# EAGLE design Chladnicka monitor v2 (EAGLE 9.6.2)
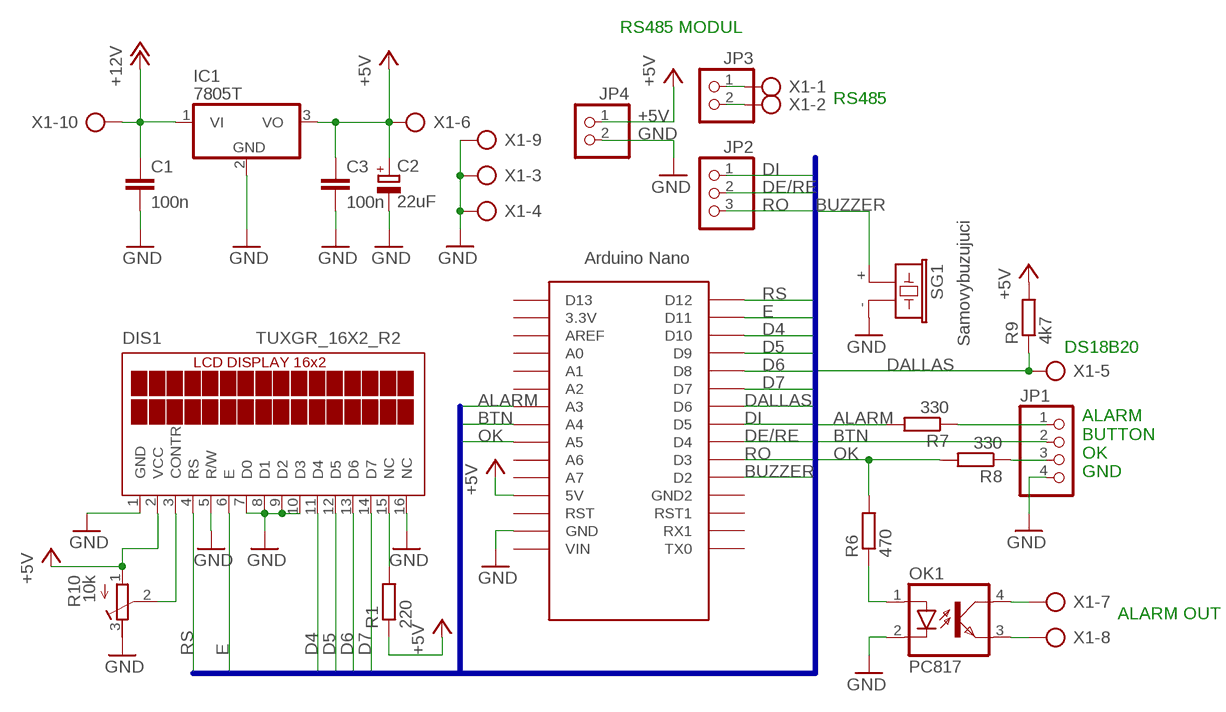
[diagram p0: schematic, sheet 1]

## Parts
C1  100n  C-EU050-024X044  [C050-024X044]
C2  22uF  CPOL-EUE2,5-6E  [E2,5-6E]
C3  100n  C-EU050-024X044  [C050-024X044]
DIS1  TUXGR_16X2_R2  [TUXGR_16X2_R2]
IC1  7805T  [TO220H]
JP1  PINHD-1X4  [1X04]
JP2  PINHD-1X3  [1X03]
JP3  PINHD-1X2  [1X02]
JP4  PINHD-1X2  [1X02]
OK1  PC817  [DIL04]
R1  220  R-EU_0204/7  [0204/7]
R6  470  R-EU_0204/7  [0204/7]
R7  330  R-EU_0204/7  [0204/7]
R8  330  R-EU_0204/7  [0204/7]
R9  4k7  R-EU_0204/7  [0204/7]
R10  10k  R-TRIMM3339P  [RTRIM3339P]
SG1  Samovybuzujuci  F/CM12P  [F/CM12P]
U$1  NANO  [NANO]
X1  AK500/10  [AK500/10]

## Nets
+5V: C2.+ C3.1 DIS1.2(VCC) IC1.3(VO) JP4.1 R1.1 R9.2 R10.1(A) U$1.5V X1.6
+12V: C1.1 IC1.1(VI) X1.10
ALARM: R7.2 U$1.A3
BTN: JP1.2 U$1.A4
BUZZER: SG1.+ U$1.D2
D4: DIS1.11(D4) U$1.D10
D5: DIS1.12(D5) U$1.D9
D6: DIS1.13(D6) U$1.D8
D7: DIS1.14(D7) U$1.D7
DALLAS: R9.1 U$1.D6 X1.5
DE/RE: JP2.2 U$1.D4
DI: JP2.1 U$1.D5
E: DIS1.6(E) U$1.D11
GND: C1.2 C2.- C3.2 DIS1.1(GND) DIS1.5(R/W) DIS1.7(D0) DIS1.8(D1) DIS1.9(D2) DIS1.10(D3) DIS1.16(NC) IC1.2(GND) JP1.4 JP4.2 OK1.2(C) R10.3(E) SG1.- U$1.GND X1.3 X1.4 X1.9
N$1: OK1.1(A) R6.1
N$2: JP1.3 R8.1
N$3: JP1.1 R7.1
N$4: JP3.2 X1.2
N$5: JP3.1 X1.1
N$6: DIS1.3(CONTR) R10.2(S)
N$7: OK1.4(COL) X1.7
N$8: OK1.3(EMIT) X1.8
N$10: DIS1.15(NC) R1.2
OK: R6.2 R8.2 U$1.A5
RO: JP2.3 U$1.D3
RS: DIS1.4(RS) U$1.D12
Unconnected: U$1.3.3V U$1.A0 U$1.A1 U$1.A2 U$1.A6 U$1.A7 U$1.AREF U$1.D13 U$1.GND1(GND2) U$1.ICSP1 U$1.ICSP2 U$1.ICSP3 U$1.ICSP4 U$1.ICSP5 U$1.ICSP6 U$1.RAW(VIN) U$1.RST U$1.RST1 U$1.RX1 U$1.TX0

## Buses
ALARM,BTN,BUZZER,D4,D5,D6,D7,DALLAS,DE/RE,DI,E,OK,RO,RS

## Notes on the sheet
- RS485 MODUL
- RS485
- DS18B20
- ALARM
  BUTTON
  OK
  GND
- ALARM OUT

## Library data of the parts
C1 C3 = rcl:C-EU: CAPACITOR, European symbol; SPICEPREFIX: C
C2 = rcl:CPOL-EU: POLARIZED CAPACITOR, European symbol; SPICEPREFIX: C
DIS1 = display-lcd:TUXGR_16X2_R2: Tuxgraphics LCD display 16x2 characters reflective, without background light Source: tuxgr_12x2_r2.pdf; OC_FARNELL: unknown; OC_NEWARK: unknown
IC1 = linear:78*: Positive VOLTAGE REGULATOR Source: http://cache.national.com/ds/LM/LM78L05.pdf http://www.fairchildsemi.com/ds/LM/LM7805.pdf
JP1 = pinhead:PINHD-1X4: PIN HEADER
JP2 = pinhead:PINHD-1X3: PIN HEADER
JP3 JP4 = pinhead:PINHD-1X2: PIN HEADER
OK1 = optocoupler:PC817: SHARP OPTO COUPLER; MPN: PC817X4J000F; OC_FARNELL: 9707727; OC_NEWARK: 97K7059
R1 R6-R9 = rcl:R-EU_: RESISTOR, European symbol; SPICEPREFIX: R
R10 = rcl:R-TRIMM: Trimm resistor; SPICEMODEL: X; SPICEPREFIXL: POT
SG1 = buzzer:F/CM12P: BUZZER; OC_FARNELL: unknown; OC_NEWARK: unknown
U$1 = Arduino-clone:NANO: Arduino Nano
X1 = con-ptr500:AK500/10: CONNECTOR; OC_FARNELL: unknown; OC_NEWARK: unknown

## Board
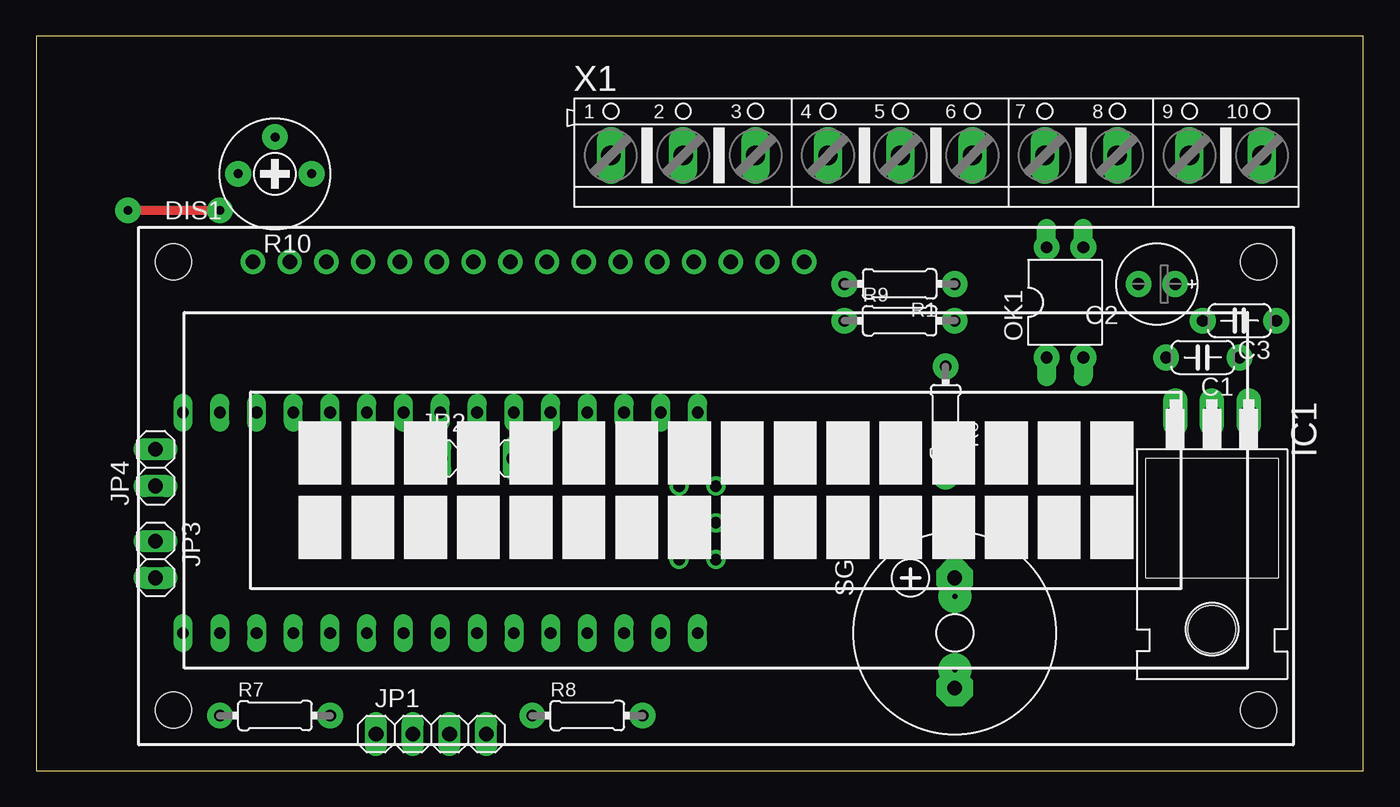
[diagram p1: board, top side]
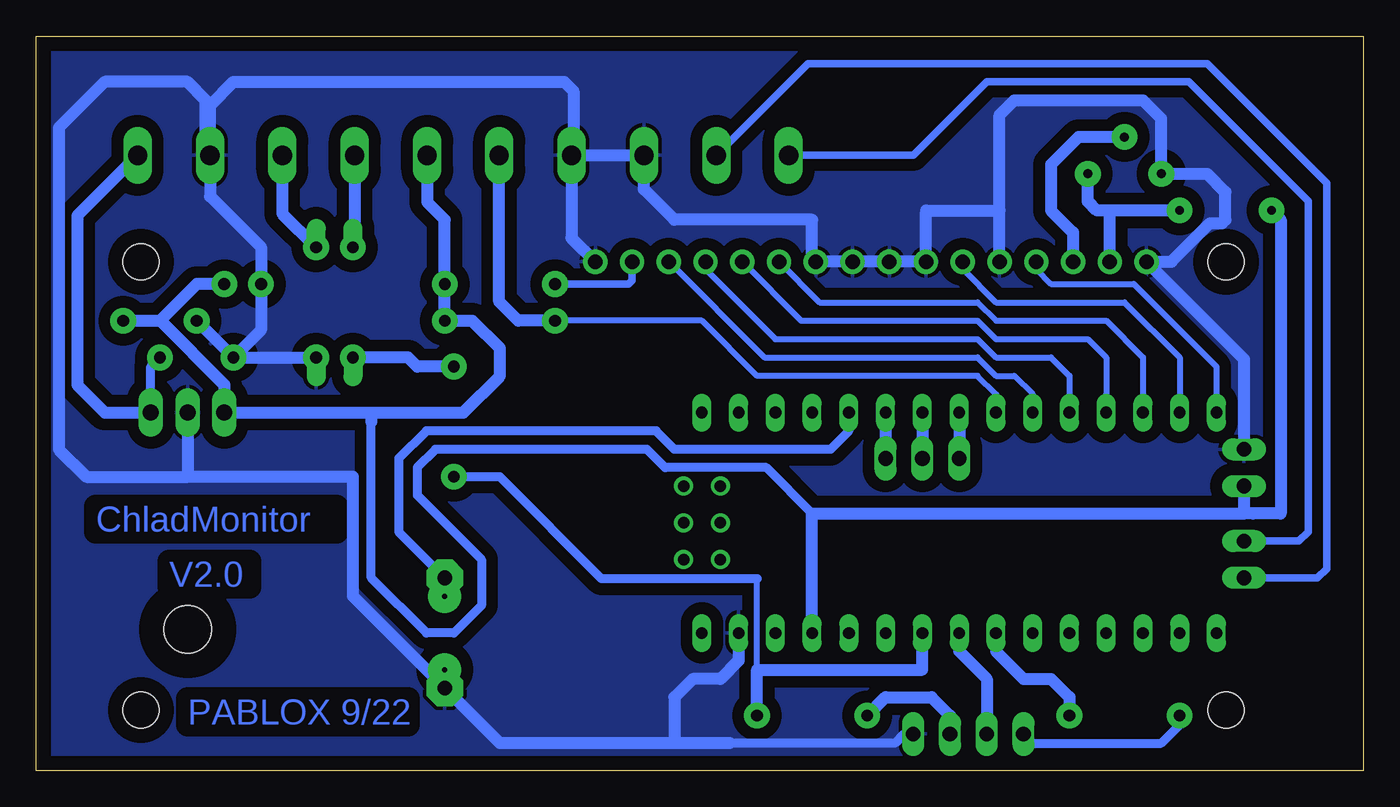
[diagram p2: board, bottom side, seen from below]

Size 91.75 x 50.79 mm. Coordinates in mm from the lower left corner, seen from the top.
Outline: 0,0 91.75,0 91.75,50.79 0,50.79 0,0
Copper layers (1*16): Top 0.035mm / dielectric 1.5mm / Bottom 0.035mm
Design rules "default": minimum track width 6mil, minimum drill 0.35mm, track to track 6mil, track to pad 6mil, pad to pad 6mil, via to via 6mil, smd to smd 6mil, copper to edge 40mil, drill to drill 6mil, minimum pad ring 10mil, minimum via ring 8mil, stop-mask expansion 4mil, vias tented up to drill 0mil, thermal gap 10mil

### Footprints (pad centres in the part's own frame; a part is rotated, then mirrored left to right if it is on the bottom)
C050-024X044 = drill 0.813 octagon: 1 -2.54,0; 2 2.54,0
E2,5-6E = drill 0.813 pad 1.575: + -1.27,0 | drill 0.813 pad 1.575 octagon: - 1.27,0
TUXGR_16X2_R2 = drill 1 pad 1.676: 1 -32,15.5; 2 -29.46,15.5; 3 -26.92,15.5; 4 -24.38,15.5; 5 -21.84,15.5; 6 -19.3,15.5; 7 -16.76,15.5; 8 -14.22,15.5; 9 -11.68,15.5; 10 -9.14,15.5; 11 -6.6,15.5; 12 -4.06,15.5; 13 -1.52,15.5; 14 1.02,15.5; 15 3.56,15.5; 16 6.1,15.5 | hole 2.5: -37.5,-15.5; 37.5,-15.5; -37.5,15.5; 37.5,15.5
TO220H = drill 1.118 long: 1 -2.54,-10.16; 2 0,-10.16; 3 2.54,-10.16 | hole 3.302: 0,4.826
1X04 = drill 1.016 long: 1 -3.81,0; 2 -1.27,0; 3 1.27,0; 4 3.81,0
1X03 = drill 1.016 long: 1 -2.54,0; 2 0,0; 3 2.54,0
1X02 = drill 1.016 long: 1 -1.27,0; 2 1.27,0
DIL04 = drill 0.813 offset: 1 -1.27,-3.81; 2 1.27,-3.81; 3 1.27,3.81; 4 -1.27,3.81
0204/7 = drill 0.813 octagon: 1 -3.81,0; 2 3.81,0
RTRIM3339P = drill 0.61: 1 -2.54,0; 2 0,-2.54; 3 2.54,0
F/CM12P = drill 1.016 pad 2.54 octagon: + 3.81,0; - -3.81,0
NANO = drill 0.8 long: 3.3V -10.16,24.13; 5V -10.16,-1.27; A0 -10.16,19.05; A1 -10.16,16.51; A2 -10.16,13.97; A3 -10.16,11.43; A4 -10.16,8.89; A5 -10.16,6.35; A6 -10.16,3.81; A7 -10.16,1.27; AREF -10.16,21.59; D2 5.08,1.27; D3 5.08,3.81; D4 5.08,6.35; D5 5.08,8.89; D6 5.08,11.43; D7 5.08,13.97; D8 5.08,16.51; D9 5.08,19.05; D10 5.08,21.59; D11 5.08,24.13; D12 5.08,26.67; D13 -10.16,26.67; GND -10.16,-6.35; GND1 5.08,-1.27; RAW -10.16,-8.89; RST -10.16,-3.81; RST1 5.08,-3.81; RX1 5.08,-6.35; TX0 5.08,-8.89 | drill 0.8: ICSP1 -5.08,-10.16; ICSP2 -5.08,-7.62; ICSP3 -2.54,-10.16; ICSP4 -2.54,-7.62; ICSP5 0,-10.16; ICSP6 0,-7.62
AK500/10 = drill 1.321 long: 1 -22.504,0; 2 -17.501,0; 3 -12.497,0; 4 -7.493,0; 5 -2.489,0; 6 2.489,0; 7 7.493,0; 8 12.497,0; 9 17.501,0; 10 22.504,0

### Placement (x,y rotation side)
C1  80.65,28.57 180 top
C2  77.47,33.66 180 top
C3  83.19,31.12 180 top
DIS1  46.99,19.68 0 top
IC1  81.28,14.6 180 top
JP1  27.3,2.54 0 top
JP2  30.48,21.59 0 top
JP3  8.26,14.6 270 top
JP4  8.26,20.95 90 top
OK1  71.12,32.38 0 top
R1  59.69,33.66 180 top
R6  62.87,24.13 270 top
R7  16.51,3.81 0 top
R8  38.1,3.81 0 top
R9  59.69,31.12 0 top
R10  16.51,41.27 180 top
SG1  63.5,9.52 90 top
U$1  36.83,19.68 90 top
X1  62.23,42.54 0 top

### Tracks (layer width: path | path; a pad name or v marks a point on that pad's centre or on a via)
+5V  (via drill 0.6 pad 1.78)
  Top 0.61: v12.7,38.73 v6.35,38.73
  Bottom 0.61: 84.92,31.12 C3.1 | 38.1,17.78 41.27,20.95 48.26,20.95 49.53,22.23 64.14,22.23 65.41,20.95 65.41,19.05 60.96,14.6 60.96,11.43 62.87,9.52 64.77,9.52 68.58,13.34 68.58,24.13
  Bottom 0.813: v6.35,38.73 5.71,38.1 5.71,17.78 7.62,17.78 8.26,17.78 | C3.1 83.19,31.12 | 83.19,31.12 78.74,26.67 IC1.3 68.58,24.77 | v12.7,38.73 17.78,38.73 | 17.78,38.73 18.41,38.73 19.05,39.37 R10.1 | DIS1.2 17.53,38.48 17.78,38.73 | C2.+ 80.65,33.66 83.19,31.12 | 68.58,24.77 62.23,24.77 59.69,27.3 59.69,29.21 61.59,31.12 R9.2 R1.1 63.5,38.1 64.72,39.32 X1.6 | 68.58,24.77 68.58,24.13 | JP4.1 8.26,17.78 | U$1.5V 38.1,17.78 8.26,17.78
+12V
  Bottom 0.61: IC1.1 83.82,27.94 C1.1
  Bottom 0.813: X1.10 88.9,38.38 88.9,26.67 87,24.77 IC1.1
ALARM
  Bottom 0.406: U$1.A3 25.4,8.89
  Bottom 0.813: U$1.A3 25.4,8.25 23.5,6.35 21.59,6.35 20.32,5.08 R7.2
BTN
  Bottom 0.813: U$1.A4 27.94,8.25 26.04,6.35 JP1.2
BUZZER
  Bottom 0.61: U$1.D2 35.56,23.49 36.83,22.23 47.62,22.23 48.89,23.49 64.77,23.49 66.67,21.59 66.67,16.51 SG1.+
D4
  Bottom 0.406: DIS1.11 37.59,32.38 26.67,32.38 25.4,31.12 17.78,31.12 15.24,28.57 U$1.D10
D5
  Bottom 0.406: DIS1.12 38.86,31.12 26.67,31.12 25.4,29.84 19.05,29.84 17.78,28.57 U$1.D9 17.78,26.03
D6
  Bottom 0.406: DIS1.13 45.47,34.67 40.64,29.84 26.67,29.84 25.4,28.57 21.59,28.57 20.32,27.3 U$1.D8
D7
  Bottom 0.406: DIS1.14 41.4,28.57 26.67,28.57 25.4,27.3 24.13,27.3 22.86,26.03 U$1.D7
DALLAS
  Bottom 0.406: U$1.D6 25.4,26.03 26.67,27.3 41.91,27.3 45.72,31.12 R9.1
  Bottom 0.813: R9.1 58.42,31.12 59.74,32.44 X1.5
DE/RE
  Bottom 0.813: U$1.D4 JP2.2
DI
  Bottom 0.813: U$1.D5 JP2.1
E
  Bottom 0.406: 27.69,34.67 25.4,32.38 16.51,32.38 12.7,28.57 U$1.D11
  Bottom 0.61: DIS1.6 27.69,34.67
GND
  Bottom 0.61: JP1.4 31.75,2.54 32.38,1.9 43.81,1.9
  Bottom 0.813: DIS1.5 25.15,38.73 | 25.15,38.73 25.15,45.34 24.13,46.35 15.24,46.35 13.97,45.09 R10.3 10.79,41.27 9.53,40 9.53,38.1 9.77,37.86 10.6,37.86 13.27,35.18 DIS1.1 | 30.23,38.63 DIS1.7 DIS1.8 DIS1.9 DIS1.10 38.1,35.43 38.1,38.1 47.62,38.1 49.73,40.21 X1.3 X1.4 | 30.23,38.73 25.15,38.73 | X1.4 54.74,36.83 DIS1.16 | SG1.- 59.69,1.9 47.62,1.9 | SG1.- 64.14,6.35 | 43.81,1.9 47.62,1.9 | C1.2 76.2,30.48 C2.- 76.2,36.2 79.73,39.73 X1.9 79.73,46 78.11,47.62 55.24,47.62 54.61,46.99 54.61,42.67 X1.4 | C1.2 C3.2 | IC1.2 81.28,20.32 | 80.01,42.82 80.01,46.35 81.28,47.62 87,47.62 90.17,44.45 90.17,22.23 88.27,20.32 81.28,20.32 | C1.2 OK1.2 | SG1.- 69.85,12.06 69.85,20.32 81.28,20.32 | U$1.GND 43.18,7.62 44.45,6.35 46.35,6.35 47.62,5.08 47.62,1.9 | 14.36,35.18 DIS1.1 | DIS1.1 8.26,28.45 JP4.2
  pour Bottom (isolate 0.813): 0,50.8 92.08,50.8 92.08,0 0,0
N$1
  Bottom 0.813: R6.1 65.41,27.94 66.04,28.57 OK1.1
N$2
  Bottom 0.406: 28.57,3.81 JP1.3
  Bottom 0.813: R8.1 33.02,5.08 29.84,5.08 28.57,3.81
N$3
  Bottom 0.61: JP1.1 22.86,1.9 13.97,1.9 12.7,3.17 R7.1
N$4
  Bottom 0.508: X1.2 38.38,48.9 10.79,48.9 2.54,40.64 2.54,13.97 3.18,13.34 JP3.2
N$5
  Bottom 0.508: X1.1 31.11,42.54 26.04,47.62 12.07,47.62 3.81,39.37 3.81,16.51 4.45,15.88 JP3.1 6.99,15.88
N$6
  Bottom 0.813: R10.2 19.68,43.82 21.59,41.91 21.59,38.73 20.07,37.21 DIS1.3
N$7
  Bottom 0.61: X1.7 69.85,42.42
  Bottom 0.813: X1.7 69.72,36.32 OK1.4
N$8
  Bottom 0.813: X1.8 74.73,38.53 OK1.3
N$9  (via drill 0.35 pad 1.78)
  other vias: 16.51,43.82
N$10
  Bottom 0.508: DIS1.15 50.55,33.91 50.8,33.66 R1.2
N$11  (via drill 0.35 pad 1.78)
  other vias: 19.05,41.27
N$12  (via drill 0.35 pad 1.78)
  other vias: 63.5,31.12
N$13  (via drill 0.35 pad 1.78)
  other vias: 63.5,33.66
N$14  (via drill 0.35 pad 1.78)
  other vias: 55.88,33.66
N$15  (via drill 0.35 pad 1.78)
  other vias: 55.88,31.12
N$16  (via drill 0.35 pad 1.78)
  other vias: 62.87,27.94
N$17  (via drill 0.35 pad 1.78)
  other vias: 78.74,33.66
N$18  (via drill 0.35 pad 1.78)
  other vias: 13.97,41.27
N$19  (via drill 0.35 pad 1.78)
  other vias: 85.73,31.12
N$20  (via drill 0.35 pad 1.78)
  other vias: 34.29,3.81
N$21  (via drill 0.35 pad 1.78)
  other vias: 80.65,31.12
N$22  (via drill 0.35 pad 1.78)
  other vias: 78.11,28.57
N$23  (via drill 0.35 pad 1.78)
  other vias: 41.91,3.81
N$25  (via drill 0.35 pad 1.78)
  other vias: 62.87,20.32
N$26  (via drill 0.35 pad 1.78)
  other vias: 83.19,28.57
N$35  (via drill 0.35 pad 1.78)
  other vias: 72.39,28.57
N$36  (via drill 0.35 pad 1.78)
  other vias: 69.85,36.2
N$37  (via drill 0.35 pad 1.78)
  other vias: 72.39,36.2
N$38  (via drill 0.35 pad 1.78)
  other vias: 69.85,28.57
N$39  (via drill 0.35 pad 1.78)
  other vias: 12.7,3.81
N$40  (via drill 0.35 pad 1.78)
  other vias: 20.32,3.81
N$41  (via drill 0.35 pad 1.78)
  other vias: 76.2,33.66
N$42  (via drill 0.35 pad 2.29)
  other vias: 63.5,12.06
N$43  (via drill 0.35 pad 2.29)
  other vias: 63.5,6.98
OK
  Bottom 0.406: 41.91,6.98 41.91,13.28
  Bottom 0.61: 41.91,13.28 52.65,13.28 59.69,20.32 R6.2
  Bottom 0.813: R8.2 41.91,6.98 30.48,6.98 U$1.A5
RO
  Bottom 0.813: U$1.D3 JP2.3
RS
  Bottom 0.406: U$1.D12 10.16,27.94 15.88,33.66 21.59,33.66 22.61,34.67
  Bottom 0.61: DIS1.4 22.61,34.67

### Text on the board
Bottom: ChladMonitor | V2.0 | PABLOX 9/22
